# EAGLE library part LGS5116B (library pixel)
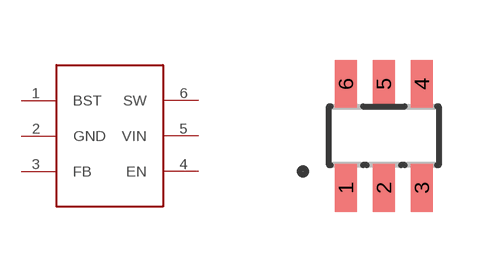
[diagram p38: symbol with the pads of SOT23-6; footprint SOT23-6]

Designator prefix -

## LGS5116B  [SOT23-6]
1  BST
2  GND
3  FB
4  EN
5  VIN
6  SW

## Footprint SOT23-6 (pad centres in mm)
6-Lead Small Outline Transistor Package SOT-23-6 Source: http://www.analog.com/UploadedFiles/Data_Sheets/346131962AD8067_a.pdf
smd 0.55 x 1.2: 1 -0.95,-1.3; 2 0,-1.3; 3 0.95,-1.3; 4 0.95,1.3; 5 0,1.3; 6 -0.95,1.3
